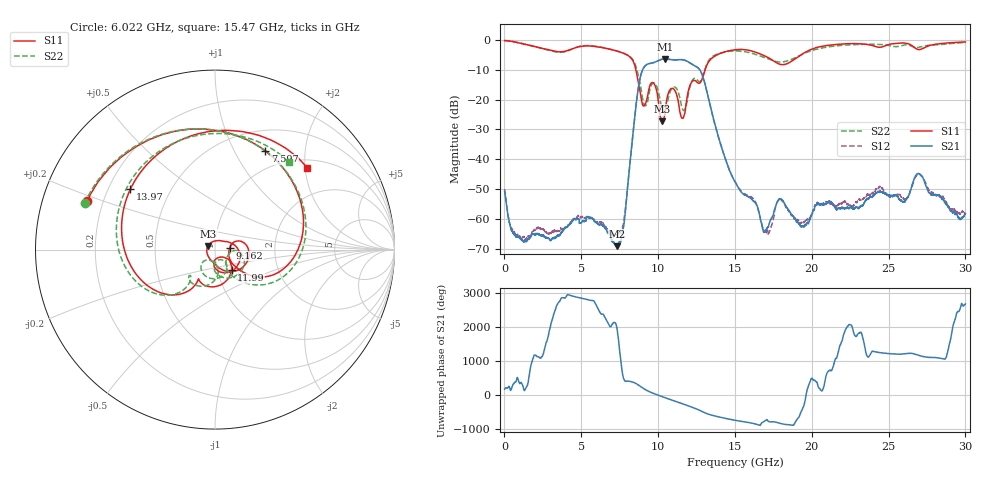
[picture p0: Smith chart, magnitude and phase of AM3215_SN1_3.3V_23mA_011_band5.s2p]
!Agilent Technologies,E8364B,MY43040894,A.07.50.67
!Agilent E8364B: A.07.50.67
!Date: Tuesday, May 25, 2021 15:24:05
!Correction: S11(Full 2 Port(1,2))
!S21(Full 2 Port(1,2))
!S12(Full 2 Port(1,2))
!S22(Full 2 Port(1,2))
!S2P File: Measurements: S11, S21, S12, S22:
# Hz S  dB  R 50
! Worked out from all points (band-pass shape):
!   6401 points, 10 MHz to 30 GHz, reference 50 ohm
!   highest |S21| = -6.40 dB at 10.43 GHz (marker M1); lowest = -69.0 dB at 7.334 GHz (marker M2)
!   |S21| within 3 dB of the highest: 9.058 GHz to 12.61 GHz (3.548 GHz wide, 32.8 % of centre)
!   lowest |S11| = -27.2 dB at 10.27 GHz (marker M3), VSWR 1.09, Z = 46.3 + j1.94 ohm
!   |S11| at or under -10 dB: 8.55 GHz to 13.06 GHz (4.512 GHz wide, 41.8 % of centre)
!   |S22| runs from -24.3 to -0.3 dB; largest |S21 - S12| = 0.005
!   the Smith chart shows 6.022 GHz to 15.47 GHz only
!   S11 on the Smith chart (normalised r, x): 6.022 GHz: 0.14, +0.18; 7.597 GHz: 0.75, +1.34; 9.162 GHz: 1.18, +0.03; 11.99 GHz: 1.17, -0.27; 13.97 GHz: 0.29, +0.30; 15.47 GHz: 1.18, +2.05
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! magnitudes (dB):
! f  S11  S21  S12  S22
! 10 MHz  -0.3  -50.7  -50.0  -0.3
! 1.219 GHz  -1.4  -67.2  -66.0  -1.4
! 5.01 GHz  -2.2  -61.0  -59.4  -2.1
! 6.022 GHz  -2.4  -61.2  -61.1  -2.3
! 7.334 GHz  -3.8  -69.0  -65.2  -3.8
! 7.597 GHz  -4.2  -66.8  -64.2  -4.3
! 8.665 GHz  -12.9  -17.8  -17.8  -11.0
! 9.162 GHz  -21.6  -8.7  -8.7  -22.1
! 10.01 GHz  -20.2  -7.0  -7.0  -17.2
! 10.27 GHz  -27.2  -6.5  -6.5  -23.5
! 10.43 GHz  -25.2  -6.4  -6.4  -24.2
! 11.99 GHz  -16.7  -7.5  -7.5  -17.6
! 12.85 GHz  -13.3  -11.5  -11.5  -13.1
! 13.97 GHz  -4.7  -33.3  -33.4  -4.6
! 15.01 GHz  -3.4  -47.5  -47.4  -3.8
! 15.47 GHz  -3.3  -51.3  -51.0  -3.9
! 17.08 GHz  -5.8  -63.2  -64.3  -6.2
! 17.88 GHz  -8.1  -53.3  -53.2  -7.5
! 20 GHz  -3.2  -58.5  -58.3  -3.6
! 25 GHz  -1.6  -52.0  -52.2  -1.9
! 26.98 GHz  -3.3  -44.8  -44.9  -2.5
! 30 GHz  -0.7  -58.1  -58.1  -0.9
